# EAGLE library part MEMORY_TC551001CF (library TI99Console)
MEMORY
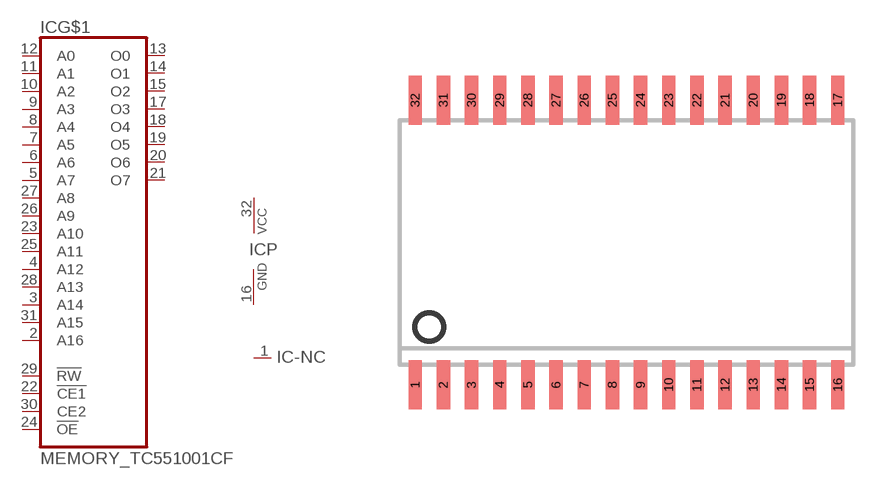
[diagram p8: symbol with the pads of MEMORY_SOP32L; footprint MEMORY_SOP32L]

Designator prefix IC; gates -NC=MEMORY_NC G$1=MEMORY_1001 P=MEMORY_PWRN

## MEMORY_TC551001CF  [MEMORY_SOP32L]
1  -NC:NC  nc
2  G$1:A16  in
3  G$1:A14  in
4  G$1:A12  in
5  G$1:A7  in
6  G$1:A6  in
7  G$1:A5  in
8  G$1:A4  in
9  G$1:A3  in
10  G$1:A2  in
11  G$1:A1  in
12  G$1:A0  in
13  G$1:O0  hiz
14  G$1:O1  hiz
15  G$1:O2  hiz
16  P:GND  pwr
17  G$1:O3  hiz
18  G$1:O4  hiz
19  G$1:O5  hiz
20  G$1:O6  hiz
21  G$1:O7  hiz
22  G$1:!CE1  in
23  G$1:A10  in
24  G$1:!OE  in
25  G$1:A11  in
26  G$1:A9  in
27  G$1:A8  in
28  G$1:A13  in
29  G$1:!RW  in
30  G$1:CE2  in
31  G$1:A15  in
32  P:VCC  pwr

## Footprint MEMORY_SOP32L (pad centres in mm)
Small Outline Package large
smd 0.6 x 2.2: 1 -9.525,-6.416; 2 -8.255,-6.416; 3 -6.985,-6.416; 4 -5.715,-6.416; 5 -4.445,-6.416; 6 -3.175,-6.416; 7 -1.905,-6.416; 8 -0.635,-6.416; 9 0.635,-6.416; 10 1.905,-6.416; 11 3.175,-6.416; 12 4.445,-6.416; 13 5.715,-6.416; 14 6.985,-6.416; 15 8.255,-6.416; 16 9.525,-6.416; 17 9.525,6.416; 18 8.255,6.416; 19 6.985,6.416; 20 5.715,6.416; 21 4.445,6.416; 22 3.175,6.416; 23 1.905,6.416; 24 0.635,6.416; 25 -0.635,6.416; 26 -1.905,6.416; 27 -3.175,6.416; 28 -4.445,6.416; 29 -5.715,6.416; 30 -6.985,6.416; 31 -8.255,6.416; 32 -9.525,6.416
